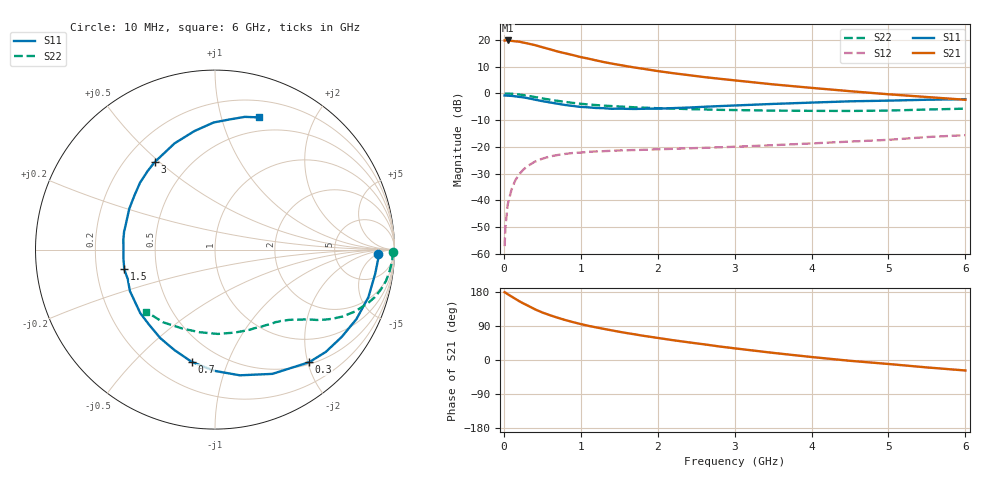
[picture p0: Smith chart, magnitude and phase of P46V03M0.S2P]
! SIEMENS Small Signal Semiconductors
! BFP182
! Si NPN RF Bipolar Junction Transistor in SOT143
! VCE = 6 V  IC = 3 mA
! Common Emitter S-Parameters:  March  1996
# GHz  S  MA  R  50
!  f  S11  S21  S12  S22
! GHz  MAG  ANG  MAG  ANG  MAG  ANG  MAG  ANG
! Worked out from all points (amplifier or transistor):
!   36 points, 10 MHz to 6 GHz, reference 50 ohm
!   highest |S21| = 19.7 dB at 50 MHz (marker M1)
!   |S21| within 3 dB of that: start of sweep to 561.9 MHz
!   unconditionally stable (mu >= 1): 1.963 GHz to 5.86 GHz
!   at 250 MHz: K = 0.16, MSG = 23.8 dB, |S12| = -28.6 dB
!   at 1.4 GHz: K = 0.78, MSG = 16.3 dB, |S12| = -21.5 dB
!   at 6 GHz: K = 0.98, MSG = 6.6 dB, |S12| = -15.6 dB
!   S11 on the Smith chart (normalised r, x): 10 MHz: 19, -6; 300 MHz: 0.53, -2.03; 700 MHz: 0.36, -0.75; 1.5 GHz: 0.32, -0.10; 3 GHz: 0.32, +0.48; 6 GHz: 0.36, +1.33
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0.01  0.9096 -1.6  9.674 178.8  0.0014 77.0  0.9942 -0.7
0.02  0.9099 -3.6  9.687 177.9  0.0031 81.2  0.988 -1.3
0.05  0.9025 -8.7  9.694 173.7  0.0084 87.9  0.9898 -3.5
0.1  0.8947 -17.3  9.519 167.5  0.016 78.9  0.9801 -7.0
0.2  0.8573 -34.6  9.208 155.2  0.0309 71.2  0.9502 -13.6
0.25  0.8403 -42.7  8.865 149.7  0.0371 66.1  0.9277 -16.7
0.3  0.8179 -50.1  8.571 144.8  0.043 62.6  0.9034 -19.2
0.4  0.7627 -65.2  7.964 134.2  0.0526 55.2  0.8536 -23.8
0.5  0.714 -78.8  7.257 125.4  0.0601 49.3  0.8034 -27.6
0.6  0.6749 -90.6  6.631 118.2  0.0662 44.4  0.7595 -30.5
0.7  0.6384 -101.8  6.017 111.5  0.0705 40.2  0.7228 -32.7
0.9  0.58 -121.6  5.157 99.9  0.077 34.5  0.6614 -36.1
1.1  0.5466 -139.6  4.433 90.1  0.0808 30.2  0.6192 -39.0
1.3  0.5272 -154.2  3.827 82.1  0.0831 27.5  0.5886 -41.4
1.5  0.5173 -167.7  3.391 74.5  0.0857 25.6  0.5668 -43.7
1.8  0.5138 173.7  2.884 64.3  0.088 24.1  0.5404 -47.4
2.2  0.5291 154.6  2.374 52.2  0.0919 22.7  0.5188 -53.1
3  0.5921 124.6  1.744 30.8  0.1005 22.2  0.4867 -66.7
3.5  0.6335 110.8  1.468 18.8  0.1075 21.9  0.4752 -76.6
4.5  0.7084 90.6  1.095 -2.1  0.1255 20.9  0.4681 -100.3
5.5  0.7581 77.3  0.852 -19.6  0.1524 18.4  0.4975 -125.5
6  0.7771 71.4  0.757 -27.7  0.1655 14.8  0.5166 -138.1
